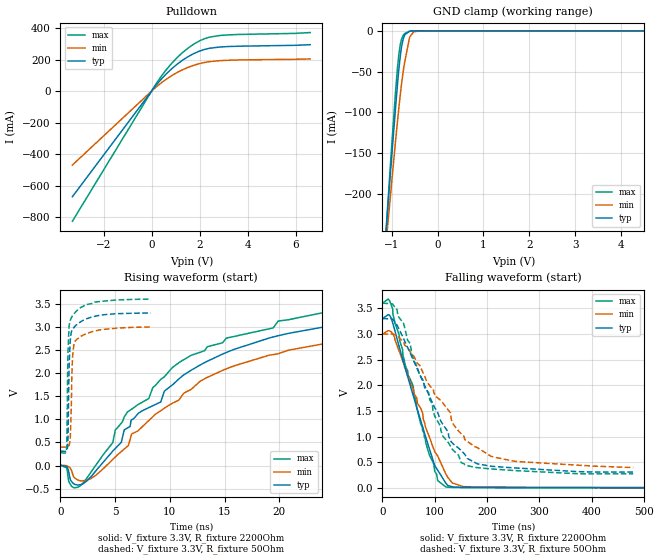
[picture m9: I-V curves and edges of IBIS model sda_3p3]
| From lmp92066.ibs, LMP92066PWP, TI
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|   sda_3p3 Model
[Model]   sda_3p3
Model_type   I/O_open_drain
Polarity   Non-Inverting
Vinl = 0.99
Vinh = 2.31
Vmeas = 1.65
Vref = 3.3
Cref = 100pF
Rref = 2200
|   typ   min   max
|   (nom PVT)   (fast PVT)   (slow PVT)
C_comp   1.263e-12   1.138e-12   1.263e-12
[Model spec]
|subparameter
Vinl   0.99   0.9   1.08
Vinh   2.31   2.1   2.52
| Where nom  PVT is Nominal Process, 3.3V, 25C
|   Fast PVT is Strong Process,  3.6V, -25C
|   Slow PVT is Weak Process,   3V, 125C
[Voltage Range]   3.3   3   3.6
|Junction Temperature
[Temperature Range]   25   125   -25
[Pullup Reference]   3.3   3   3.6
[Pulldown Reference]   0   0   0
[Power Clamp Reference]   3.3   3   3.6
[GND Clamp Reference]   0   0   0
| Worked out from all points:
|   slope of the pulldown table from 0 to 0.495 V, typ, clamps not added: 5.45 ohm
|   GND clamp passes 1 mA (typ) near -0.62 V on its own axis
|   falling waveform, V_fixture 3.3V, R_fixture 2200Ohm: 20-80 % time 57.8ns typ, 64.7ns min, 54.5ns max; typ from 3.3 V to 0.007 V
|   rising waveform, V_fixture 3.3V, R_fixture 2200Ohm: 20-80 % time 11.7ns typ, 12.8ns min, 12.5ns max; typ from 0.007 V to 3.29 V
|   falling waveform, V_fixture 3.3V, R_fixture 50Ohm: 20-80 % time 81.3ns typ, 96.5ns min, 74.7ns max; typ from 3.3 V to 0.314 V
|   rising waveform, V_fixture 3.3V, R_fixture 50Ohm: 20-80 % time 183ps typ, 209ps min, 164ps max; typ from 0.314 V to 3.3 V
[Pulldown]
|   Voltage   I(typ)   I(min)   I(max)
-3.3V     -669.9mA   -469.2mA   -825.6mA
189mV     37.64mA    26.03mA    46.69mA
462mV     85.57mA    59.23mA    106.2mA
836.4mV   141.7mA    98.01mA    176.1mA
1.251V    192.1mA    132.6mA    239.4mA
1.5V      216.8mA    149.4mA    270.8mA
1.772V    239.1mA    164.5mA    299.5mA
2.19V     263.5mA    181.2mA    331.4mA
2.832V    279.5mA    193.1mA    352.6mA
6.6V      294.3mA    204.1mA    371.3mA
[GND Clamp]
|   Voltage   I(typ)   I(min)   I(max)
-3.3V     -1.762A    -1.414A    -1.847A
-1.374V   -440.4mA   -410.4mA   -458.7mA
-1.049V   -190.8mA   -216.6mA   -183mA
-915mV    -94.28mA   -135mA     -74.02mA
-844.8mV  -47.85mA   -95.36mA   -29.66mA
-792mV    -22.34mA   -68.44mA   -11.63mA
-747.6mV  -9.718mA   -49.29mA   -5.386mA
-712.8mV  -4.668mA   -37.43mA   -3.217mA
-614.4mV  -611.7uA   -9.316mA   -587.2uA
-519mV    -65.41uA   -1.036mA   -51.23uA
-330mV    -289.5nA   -7.736uA   -91.36nA
6.6V      0A         0A         0A
[POWER Clamp]
|   Voltage   I(typ)   I(min)   I(max)
-3.3V     0A         0A         0A
0V        0A         0A         0A
6.6V      0A         0A         0A
[Ramp]
R_load = 2200
|   typ   min   max
dV/dt_r   1.9756/1.16753e-08   1.79453/1.3096e-08   2.15612/1.2699e-08
dV/dt_f   1.9756/5.785e-08   1.79453/6.48707e-08   2.15612/5.48728e-08
[Falling Waveform]
V_fixture = 3.3V
V_fixture_min = 3V
V_fixture_max = 3.6V
R_fixture = 2200Ohm
|   Time   V(typ)   V(min)   V(max)
0s        3.3V       3V         3.6V
11.34ns   3.376V     3.065V     3.676V
19.45ns   3.222V     3.005V     3.49V
58.88ns   1.799V     1.925V     1.979V
77.02ns   1.185V     1.456V     1.119V
85.62ns   900.1mV    1.1V       782.2mV
105.6ns   351.7mV    628.5mV    148mV
121.2ns   98.57mV    276mV      23.33mV
154.9ns   14.75mV    29.18mV    11.64mV
846.4ns   7.329mV    9.616mV    6.458mV
[Rising Waveform]
V_fixture = 3.3V
V_fixture_min = 3V
V_fixture_max = 3.6V
R_fixture = 2200Ohm
|   Time   V(typ)   V(min)   V(max)
0s        7.329mV    9.616mV    6.458mV
548.4ps   -23.04mV   -789.9uV   -46.09mV
994.8ps   -339.1mV   -98.27mV   -441.1mV
1.778ns   -415.2mV   -326.5mV   -444.6mV
6.122ns   813.1mV    417.8mV    1.16V
10.23ns   1.746V     1.349V     2.122V
13.42ns   2.256V     1.907V     2.57V
19.89ns   2.808V     2.418V     3.126V
33.47ns   3.201V     2.875V     3.501V
53ns      3.29V      2.987V     3.59V
[Falling Waveform]
V_fixture = 3.3V
V_fixture_min = 3V
V_fixture_max = 3.6V
R_fixture = 50Ohm
|   Time   V(typ)   V(min)   V(max)
0s        3.3V       3V         3.6V
27.9ns    3.171V     2.964V     3.473V
60.01ns   2.47V      2.567V     2.482V
88.27ns   1.826V     2.023V     1.858V
115.1ns   1.249V     1.664V     1.022V
131.3ns   903.8mV    1.364V     794.1mV
150.7ns   732.8mV    1.059V     497.5mV
181.4ns   474mV      790mV      400.2mV
250.3ns   395.7mV    527mV      345.2mV
479.8ns   313.8mV    403mV      279.3mV
[Rising Waveform]
V_fixture = 3.3V
V_fixture_min = 3V
V_fixture_max = 3.6V
R_fixture = 50Ohm
|   Time   V(typ)   V(min)   V(max)
0s        313.7mV    402.1mV    279.3mV
548.4ps   317.4mV    398.6mV    324.6mV
600.7ps   337.4mV    401.1mV    790mV
646ps     390.2mV    405.9mV    1.837V
811.5ps   2.284V     450.1mV    3.051V
904.9ps   2.727V     635.4mV    3.146V
1.019ns   2.902V     1.642V     3.209V
1.171ns   2.966V     2.51V      3.265V
1.488ns   3.047V     2.729V     3.347V
8.238ns   3.298V     2.996V     3.599V
